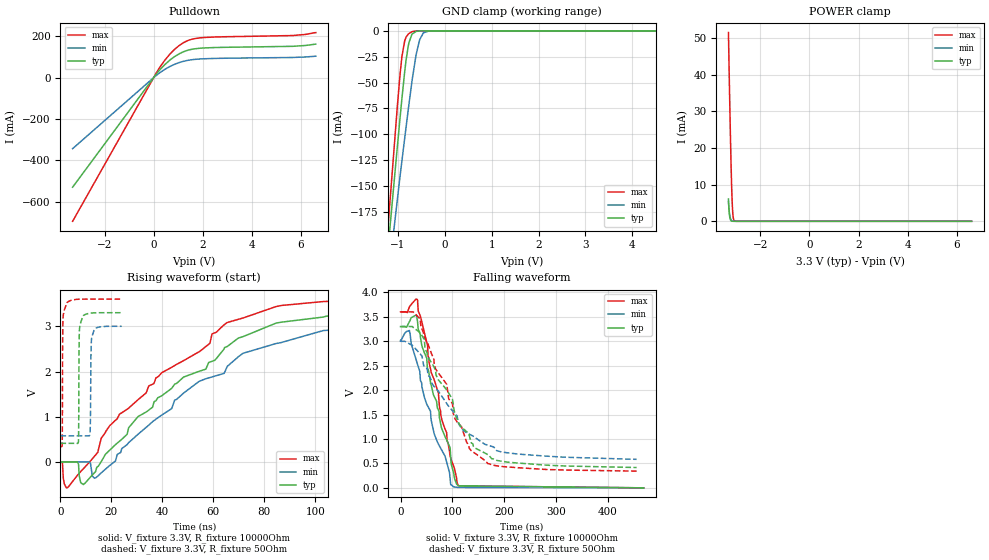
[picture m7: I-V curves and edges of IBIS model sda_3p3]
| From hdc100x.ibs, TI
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|   sda_3p3 Model
[Model]   sda_3p3
Model_type   I/O_open_drain
Polarity   Non-Inverting
Vinl = 0.99
Vinh = 2.31
Vmeas = 1.65
Vref = 3.3
Cref = 2pF
Rref = 10000
|   typ   min   max
|   (nom PVT)   (fast PVT)   (slow PVT)
C_comp   3.656e-12   3.601e-12   3.702e-12
[Model spec]
|subparameter
Vinl   0.99   0.90   1.08
Vinh   2.31   2.10   2.52
| Where nom  PVT is Nominal Process, 3.3V, 27C
|   Fast PVT is Strong Process,  3.6V, -40C
|   Slow PVT is Weak Process,   3V, 150C
[Voltage Range]   3.3   3   3.6
|Junction Temperature
[Temperature Range]   27   150   -40
[Pullup Reference]   3.3   3   3.6
[Pulldown Reference]   0   0   0
[Power Clamp Reference]   3.3   3   3.6
[GND Clamp Reference]   0   0   0
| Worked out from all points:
|   slope of the pulldown table from 0 to 0.495 V, typ, clamps not added: 7.34 ohm
|   GND clamp passes 1 mA (typ) near -0.62 V on its own axis
|   POWER clamp passes 1 mA (typ) near -3.24 V on its own axis
|   falling waveform, V_fixture 3.3V, R_fixture 10000Ohm: 20-80 % time 45.9ns typ, 50.3ns min, 42.4ns max; typ from 3.3 V to 0.002 V
|   rising waveform, V_fixture 3.3V, R_fixture 10000Ohm: 20-80 % time 41ns typ, 41.8ns min, 43ns max; typ from 0.002 V to 3.29 V
|   falling waveform, V_fixture 3.3V, R_fixture 50Ohm: 20-80 % time 83ns typ, 94.1ns min, 72.7ns max; typ from 3.3 V to 0.418 V
|   rising waveform, V_fixture 3.3V, R_fixture 50Ohm: 20-80 % time 180ps typ, 254ps min, 157ps max; typ from 0.413 V to 3.3 V
[Pulldown]
|   Voltage   I(typ)   I(min)   I(max)
-3.3V     -529mA     -342.9mA   -693.7mA
134.4mV   21.17mA    13.45mA    28.23mA
432mV     60.41mA    38.38mA    80.64mA
652.8mV   84.1mA     53.37mA    112.6mA
1.031V    114.6mA    72.51mA    154.3mA
1.442V    134.1mA    84.69mA    181.3mA
1.905V    142.3mA    90.36mA    192.5mA
5.655V    151.4mA    97.44mA    203.4mA
6.6V      162mA      103.5mA    217.8mA
[GND Clamp]
|   Voltage   I(typ)   I(min)   I(max)
-3.3V     -1.065A    -981.4mA   -1.128A
-1.381V   -296.3mA   -310mA     -290.7mA
-1.007V   -111.2mA   -162.5mA   -72.05mA
-913.2mV  -66.42mA   -126.4mA   -25.74mA
-852mV    -39.51mA   -103.8mA   -9.648mA
-776.4mV  -14.75mA   -76.39mA   -3.214mA
-699mV    -3.563mA   -49.56mA   -929.7uA
-609mV    -571.8uA   -23.07mA   -104uA
-534mV    -101.2uA   -8.759mA   -10.44uA
-453mV    -12.35uA   -1.907mA   -596.2nA
-330mV    -322nA     -97.28uA   0A
6.6V      0A         0A         0A
[POWER Clamp]
|   Voltage   I(typ)   I(min)   I(max)
-3.3V     6.079mA    5.422mA    51.48mA
-3.285V   4.075mA    3.945mA    45.96mA
-3.26V    1.908mA    2.239mA    37.15mA
-3.237V   849uA      1.253mA    29.12mA
-3.216V   393.1uA    727.4uA    22.33mA
-3.185V   120.4uA    316.3uA    13.31mA
-3.163V   52.62uA    175.5uA    8.179mA
-3.142V   22.84uA    96.55uA    4.338mA
-3.12V    9.942uA    52.54uA    1.948mA
-3.098V   4.309uA    28.13uA    761.6uA
-3.052V   706.8nA    6.22uA     80.17uA
6.6V      0A         0A         0A
[Ramp]
R_load = 10000
|   typ   min   max
dV/dt_r   1.97842/4.12082e-08   1.81097/4.18779e-08   2.15873/4.2809e-08
dV/dt_f   1.97871/4.58818e-08   1.81135/5.0703e-08   2.15892/4.26244e-08
[Falling Waveform]
V_fixture = 3.3V
V_fixture_min = 3V
V_fixture_max = 3.6V
R_fixture = 10000Ohm
|   Time   V(typ)   V(min)   V(max)
0s        3.3V       3V         3.6V
17.14ns   3.401V     3.22V      3.703V
32.81ns   3.394V     2.527V     3.843V
52.17ns   2.446V     1.681V     2.909V
58.81ns   2.116V     1.419V     2.37V
65.24ns   1.864V     1.095V     2.202V
85.73ns   1.05V      652.1mV    1.205V
96.73ns   622.9mV    66.66mV    610.4mV
112.4ns   42.62mV    9.34mV     42.82mV
468.7ns   2.071mV    2.983mV    1.698mV
[Rising Waveform]
V_fixture = 3.3V
V_fixture_min = 3V
V_fixture_max = 3.6V
R_fixture = 10000Ohm
|   Time   V(typ)   V(min)   V(max)
0s        2.049mV    2.948mV    1.682mV
2.327ns   2.049mV    2.948mV    -570.8mV
6.631ns   2.209mV    2.948mV    -295.6mV
9.006ns   -498.3mV   2.948mV    -147.5mV
13.9ns    -190.1mV   -346.6mV   163.6mV
23.19ns   459.8mV    196.8mV    1.059V
38.22ns   1.421V     976.7mV    1.881V
65.31ns   2.55V      2.091V     3.08V
103.2ns   3.204V     2.906V     3.547V
158.3ns   3.294V     3.012V     3.596V
[Falling Waveform]
V_fixture = 3.3V
V_fixture_min = 3V
V_fixture_max = 3.6V
R_fixture = 50Ohm
|   Time   V(typ)   V(min)   V(max)
0s        3.3V       3V         3.6V
37.76ns   3.177V     2.743V     3.458V
67.7ns    2.391V     2.037V     2.432V
89.11ns   2.005V     1.726V     2.119V
100ns     1.814V     1.579V     1.726V
103.9ns   1.562V     1.533V     1.442V
132.5ns   1.069V     1.101V     808.2mV
142.5ns   823.2mV    1.04V      716.5mV
168.4ns   678.9mV    874.3mV    497.8mV
455ns     417.7mV    584.9mV    344mV
[Rising Waveform]
V_fixture = 3.3V
V_fixture_min = 3V
V_fixture_max = 3.6V
R_fixture = 50Ohm
|   Time   V(typ)   V(min)   V(max)
0s        412.8mV    578.3mV    341mV
676ps     412.8mV    578.3mV    374.5mV
983ps     412.8mV    578.3mV    3.139V
2.222ns   412.8mV    578.3mV    3.492V
7.082ns   461.8mV    578.3mV    3.597V
7.425ns   2.885V     578.3mV    3.598V
8.577ns   3.197V     578.3mV    3.599V
11.65ns   3.289V     640.6mV    3.6V
13.15ns   3.297V     2.91V      3.6V
24.04ns   3.3V       3V         3.6V
